FUNCTION_BLOCK FB13
TITLE =Get Motor Parameter
//*****************************************************************************
//* maxon motor ag
//* R&D
//* all rights reserved
//*****************************************************************************
//* Summary:  Read motor parameters
//*
//* Remarks:
//*
//* Created under: STEP7 REV5.2+SP1
//*****************************************************************************
//* History:
//* 19.05.2004 | INA   first release
//*
//*
//*****************************************************************************

AUTHOR:INA
FAMILY:Configur
NAME:GMotPara
VERSION:00.01


VAR_INPUT

Read : BOOL //A rising edge start the command

  NodeID : BYTE //Adress of the maxon device

END_VAR
VAR_OUTPUT
  Done : BOOL //Data valid flag is TRUE if data were available

  Err : BOOL //Error flag is TRUE if an Error has occured, see ErrNo for more details

  ErrNo : DINT //Contains detailed error information

  MotorType : WORD //Kind of Motor

  ContinuousCurrent : WORD //Maximal Continuous Current

  PeakCurrent : WORD //Maximal Peak Current

  PolePair : BYTE //Number of Pole Pairs

  ThermalTimeConstant : WORD //Thermal Time Constant

END_VAR
VAR
  xEdgeMerker : BOOL //Edge Merker

  xEdgeFlag : BOOL //Edge Flag

  xStep : INT
END_VAR

BEGIN

NETWORK
TITLE = Activate the service function
//

// SDO Read "Get Motor Parameter"

       U    #Read
       FP   #xEdgeFlag                   // recognize a positiv edge of the Read signal
       =    #xEdgeMerker                 // and set the xEdgeMerker for one cycle to true

       L    #xStep
       L    0
       ==I
       U    #xEdgeMerker
       SPB  nstp                         // iStep = 1 -> fnc1

       L    #xStep                       // jump list
       SPL  List
       SPA  rdef
       SPA  fnc1
       SPA  fncE
List  :SPA  rdef

rdef  :NOP  0
       R    #Done                        // reset Done
       R    #Err                         // reset Error
       L    0
       T    #xStep                       // iStep = 0
       SPA  end

fnc1  :NOP  0
       CALL FC1
         NodeID:=#NodeID
         Index:=DW#16#00006402
         SubIndex:=DW#16#00000000        // MotorType
         RET_VAL:=#Done
         Err:=#Err
         ErrNo:=#ErrNo

       L    DB219.DBW10
       T    #MotorType

       L    1
       U    #Err
       SPB  fncE

       NOP  0
       CALL FC1
         NodeID:=#NodeID
         Index:=DW#16#00006410
         SubIndex:=DW#16#00000001        // Max Continuous Current
         RET_VAL:=#Done
         Err:=#Err
         ErrNo:=#ErrNo

       L    DB219.DBW10
       T    #ContinuousCurrent

       L    1
       U    #Err
       SPB  fncE

       NOP  0
       CALL FC1
         NodeID:=#NodeID
         Index:=DW#16#00006410
         SubIndex:=DW#16#00000002        // Max Peak Current
         RET_VAL:=#Done
         Err:=#Err
         ErrNo:=#ErrNo

       L    DB219.DBW10
       T    #PeakCurrent

       L    1
       U    #Err
       SPB  fncE

       NOP  0
       CALL FC1
         NodeID:=#NodeID
         Index:=DW#16#00006410
         SubIndex:=DW#16#00000003        // Pole Pair
         RET_VAL:=#Done
         Err:=#Err
         ErrNo:=#ErrNo

       L    DB219.DBB10
       T    #PolePair

       L    1
       U    #Err
       SPB  fncE

       NOP  0
       CALL FC1
         NodeID:=#NodeID
         Index:=DW#16#00006410
         SubIndex:=DW#16#00000005        // Thermal Time Constant
         RET_VAL:=#Done
         Err:=#Err
         ErrNo:=#ErrNo

       L    DB219.DBW10
       T    #ThermalTimeConstant

fncE  :NOP  0
       L    0
       T    #xStep
       SPA  end

nstp  :NOP  0
       L    #xStep
       INC            1
       T    #xStep

end   :NOP  0
END_FUNCTION_BLOCK
